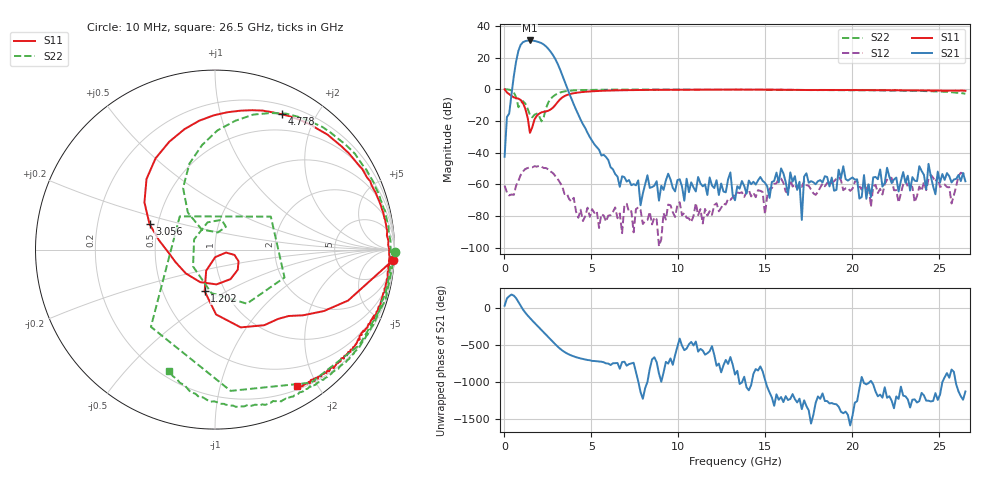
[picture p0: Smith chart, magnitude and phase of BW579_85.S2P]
!Agilent Technologies,N5242A,MY52422126,A.09.90.01
!Agilent N5242A: A.09.90.01
!Date: Wednesday, November 18, 2015 21:44:44
!Correction: S11(Full 2 Port(1,2))
!S21(Full 2 Port(1,2))
!S12(Full 2 Port(1,2))
!S22(Full 2 Port(1,2))
!S2P File: Measurements: S11, S21, S12, S22:
# Hz S  dB  R 50
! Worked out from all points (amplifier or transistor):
!   201 points, 10 MHz to 26.5 GHz, reference 50 ohm
!   highest |S21| = 30.8 dB at 1.467 GHz (marker M1)
!   |S21| within 3 dB of that: 925.8 MHz to 2.308 GHz (1.382 GHz wide, 85.5 % of centre)
!   unconditionally stable (mu >= 1): 56.96 MHz to end of sweep
!   at 4.381 GHz: K = 1211.15, MAG = -5.4 dB, |S12| = -76.0 dB
!   at 13.26 GHz: K = 10185.08, MAG = -45.1 dB, |S12| = -66.1 dB
!   at 26.5 GHz: K = 19006.44, MAG = -48.1 dB, |S12| = -53.5 dB
!   S11 on the Smith chart (normalised r, x): 10 MHz: 4, -33; 1.202 GHz: 0.80, -0.40; 3.056 GHz: 0.45, +0.15; 4.778 GHz: 0.30, +1.57; 26.5 GHz: 0.24, -1.75
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1e7  -0.07 -3.5  -42.61 30.5  -60.81 -26.1  0.04 -0.8
5.398e8  -5.15 -42.0  8.31 167.1  -66.69 -88.9  -2.03 -83.7
8.047e8  -5.97 -56.9  24.34 80.6  -57.78 -148.1  -11.38 136.7
9.3715e8  -6.81 -71.7  28.09 26.7  -54.03 165.4  -8.84 30.6
1.0696e9  -8.84 -89.0  29.72 -22.0  -51.86 126.3  -7.59 -21.9
1.20205e9  -12.41 -103.9  30.37 -63.9  -50.32 85.4  -9.12 -59.5
1.3345e9  -17.89 -112.7  30.66 -101.4  -49.75 47.3  -12.28 -94.6
1.46695e9  -27.53 -88.5  30.77 -136.4  -49.33 14.1  -16.24 -142.5
1.5994e9  -23.98 -15.1  30.66 -169.8  -49.31 -17.7  -17.74 153.8
1.73185e9  -18.98 -15.3  30.46 157.9  -48.62 -45.1  -16.05 105.1
1.99675e9  -15.43 -41.4  29.65 94.6  -48.36 -99.2  -17.00 64.4
2.26165e9  -14.24 -87.6  28.20 29.2  -49.71 -154.7  -17.47 123.3
2.3941e9  -14.01 -114.6  26.97 -3.8  -49.77 -178.0  -11.86 126.3
2.659e9  -12.74 -162.4  23.61 -68.3  -51.90 130.7  -6.03 106.6
3.05635e9  -8.15 158.8  16.11 -161.6  -56.53 59.4  -2.77 81.0
4.5133e9  -1.74 71.1  -22.09 30.1  -83.19 66.4  -0.49 34.3
4.7782e9  -1.51 63.7  -27.54 15.5  -74.73 75.0  -0.47 29.8
8.88415e9  -0.36 12.4  -70.34 -167.7  -99.05 93.3  -0.18 -6.2
1.3255e10  -0.24 -12.4  -70.08 179.7  -66.06 -24.7  -0.26 -28.4
1.77583e10  -0.50 -30.2  -58.70 -8.4  -65.64 166.8  -0.48 -48.5
2.212915e10  -0.64 -44.9  -55.29 -114.7  -55.57 -148.7  -0.84 -70.0
2.65e10  -1.02 -58.9  -58.11 -50.2  -53.52 -146.2  -2.82 -110.7
